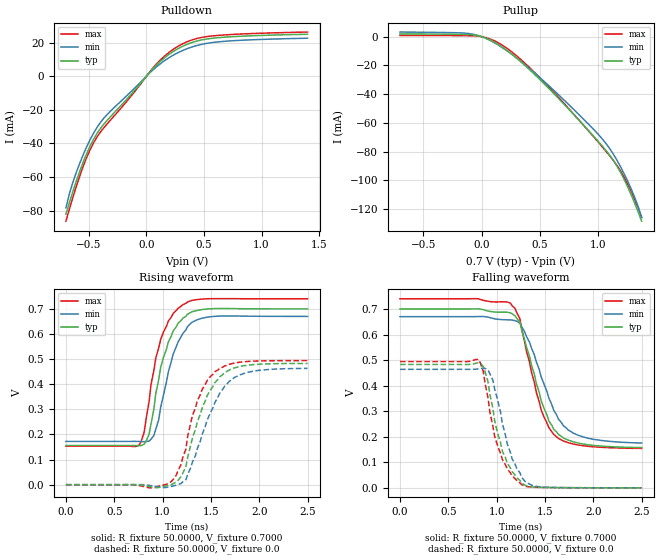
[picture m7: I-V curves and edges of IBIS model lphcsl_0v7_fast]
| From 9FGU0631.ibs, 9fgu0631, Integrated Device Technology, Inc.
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[Model]  lphcsl_0v7_fast
Model_type Output
Polarity   Non-Inverting
Enable   Active-High
Vmeas =  0.4000V
Cref =   2.0000pF
Rref =   0.0
Vref =   0.4000V
C_comp   1.1000pF   1.0000pF   1.2000pF
[Temperature Range]   25.0000   75.0000   0.0
[Voltage Range]   0.7000V   0.6700V   0.7400V
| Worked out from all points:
|   slope of the pulldown table from 0 to 0.105 V, typ, clamps not added: 13.4 ohm
|   slope of the pullup table from 0 to 0.105 V, typ, clamps not added: 28.5 ohm
|   rising waveform, R_fixture 50.0000, V_fixture 0.7000: 20-80 % time 198ps typ, 198ps min, 196ps max; typ from 0.156 V to 0.7 V
|   rising waveform, R_fixture 50.0000, V_fixture 0.0: 20-80 % time 259ps typ, 292ps min, 232ps max; typ from 0 V to 0.483 V
|   falling waveform, R_fixture 50.0000, V_fixture 0.7000: 20-80 % time 257ps typ, 294ps min, 239ps max; typ from 0.7 V to 0.158 V
|   falling waveform, R_fixture 50.0000, V_fixture 0.0: 20-80 % time 188ps typ, 200ps min, 190ps max; typ from 0.483 V to 0 V
[Pulldown]
|Voltage   I(typ)   I(min)   I(max)
-700mV    -82.14mA   -78.33mA   -86.3mA
-640mV    -68.79mA   -63.21mA   -72.24mA
-580mV    -56.64mA   -51.82mA   -59.42mA
-490mV    -41.54mA   -37.77mA   -43.75mA
-430mV    -34.05mA   -30.48mA   -36.23mA
-340mV    -26.12mA   -22.67mA   -28.22mA
-130mV    -10.53mA   -8.891mA   -11.53mA
20mV      1.656mA    1.382mA    1.825mA
200mV     13.17mA    11.18mA    14.37mA
350mV     18.87mA    16.29mA    20.4mA
530mV     22.18mA    19.61mA    23.61mA
1.4V      24.97mA    22.6mA     26.27mA
[Pullup]
|Voltage   I(typ)   I(min)   I(max)
-700mV    1.953mA    3.23mA     886.9uA
-70mV     1.182mA    1.633mA    602.4uA
80mV      -2.622mA   -2.943mA   -1.863mA
230mV     -10.45mA   -10.65mA   -8.914mA
350mV     -18.55mA   -18.18mA   -17.01mA
530mV     -32.42mA   -30.85mA   -31.3mA
830mV     -57.91mA   -54.07mA   -57.81mA
1.04V     -76.91mA   -71.94mA   -77.46mA
1.13V     -86.5mA    -82.16mA   -86.47mA
1.22V     -99.41mA   -95.52mA   -97.83mA
1.31V     -116mA     -111.9mA   -113.4mA
1.37V     -128.6mA   -126.2mA   -125.8mA
[Ramp]
| variable   typ   min   max
dV/dt_r  0.2897/0.2672n   0.2779/0.2853n   0.2965/0.2543n
dV/dt_f  0.3254/0.2576n   0.2968/0.2923n   0.3514/0.2465n
R_load = 50.0000
[Rising Waveform]
R_fixture= 50.0000
V_fixture= 0.7000
V_fixture_min= 0.6700
V_fixture_max= 0.7400
|time   V(typ)   V(min)   V(max)
0s        156.1mV    172.3mV    153.3mV
760ps     154.8mV    172.1mV    159.2mV
810ps     161.4mV    171.1mV    209.4mV
860ps     200mV      173.7mV    330.2mV
910ps     300.9mV    195.7mV    455mV
980ps     466.6mV    307.8mV    578mV
1.11ns    612.2mV    520.3mV    681.5mV
1.21ns    662.9mV    602.3mV    716.4mV
1.46ns    699.5mV    666.9mV    740.2mV
2.5ns     700mV      670mV      740mV
[Rising Waveform]
R_fixture= 50.0000
V_fixture= 0.0
V_fixture_min= 0.0
V_fixture_max= 0.0
|time   V(typ)   V(min)   V(max)
0s        0V         0V         0V
910ps     -11.41mV   -5.597mV   -11.05mV
1.09ns    314.4uV    -7.236mV   12.29mV
1.19ns    31.84mV    4.269mV    79.44mV
1.24ns    70.17mV    19.24mV    140.5mV
1.31ns    188.1mV    91.03mV    277.1mV
1.36ns    250.3mV    144.1mV    334mV
1.54ns    405.7mV    326.8mV    449.5mV
1.79ns    470mV      436.3mV    487.2mV
2.5ns     482.8mV    463.1mV    494.1mV
[Falling Waveform]
R_fixture= 50.0000
V_fixture= 0.7000
V_fixture_min= 0.6700
V_fixture_max= 0.7400
|time   V(typ)   V(min)   V(max)
0s        700mV      670mV      740mV
1.14ns    684.7mV    657.3mV    723.2mV
1.24ns    648mV      644.5mV    661.9mV
1.29ns    577.3mV    609.9mV    570mV
1.39ns    444.4mV    520.3mV    412mV
1.46ns    341.4mV    435mV      305.6mV
1.59ns    229.2mV    304.2mV    209.6mV
1.69ns    195.3mV    243.1mV    183.2mV
1.84ns    175.5mV    206.1mV    167.8mV
2.5ns     157.6mV    175.4mV    154.3mV
[Falling Waveform]
R_fixture= 50.0000
V_fixture= 0.0
V_fixture_min= 0.0
V_fixture_max= 0.0
|time   V(typ)   V(min)   V(max)
0s        483mV      463.8mV    494.2mV
810ps     489.8mV    465.6mV    502.6mV
860ps     475.7mV    468.9mV    458mV
910ps     415.3mV    461.6mV    352.4mV
980ps     261mV      385.7mV    200mV
1.01ns    213.2mV    343.8mV    164.4mV
1.11ns    95.94mV    171.3mV    73.42mV
1.26ns    18.73mV    40.64mV    12.14mV
1.46ns    1.855mV    3.446mV    1.413mV
2.5ns     49.44uV    91.67uV    35.28uV
